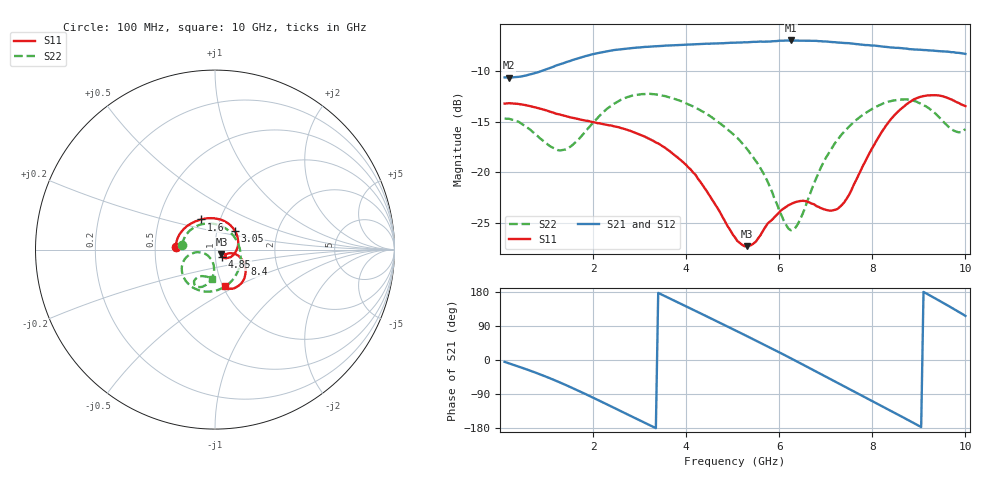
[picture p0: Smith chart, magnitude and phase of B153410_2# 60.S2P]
!  2-Port S-parameters saved by WinCal
! VAR MeasName=S-Parameters (CALIBRATED_DATA) read from VNA (N5245A)
! VAR MeasDate=2016-12-23 10:02:34
! VAR NAME=B153410_2# 60
! VAR FILENAME=B153410_2# 60.S2P
! VAR DATE=2016-12-23 10:02:34
! VAR PHYS_PORTS=1,2
# Hz S DB R 50
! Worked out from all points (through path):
!   199 points, 100 MHz to 10 GHz, reference 50 ohm
!   highest |S21| = -6.94 dB at 6.25 GHz (marker M1); lowest = -10.6 dB at 200 MHz (marker M2)
!   group delay of S21, straight-line fit = 170 ps
!   lowest |S11| = -27.3 dB at 5.3 GHz (marker M3), VSWR 1.09, Z = 53.7 - j2.54 ohm
!   |S11| at or under -10 dB: start of sweep to end of sweep
!   |S22| runs from -25.7 to -12.2 dB; largest |S21 - S12| = 0.0035
!   S11 on the Smith chart (normalised r, x): 100 MHz: 0.64, +0.02; 1.6 GHz: 0.81, +0.28; 3.05 GHz: 1.22, +0.26; 4.85 GHz: 1.08, -0.09; 8.4 GHz: 1.37, -0.23; 10 GHz: 1.02, -0.44
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1e8  -13.20 176.4  -10.60 -4.9  -10.59 -4.8  -14.69 172.4
2e8  -13.16 171.9  -10.62 -9.0  -10.62 -9.0  -14.70 163.7
9e8  -13.75 142.4  -9.96 -39.6  -9.95 -39.7  -16.78 94.6
1.6e9  -14.64 115.2  -8.82 -76.3  -8.84 -76.4  -17.13 0.2
1.75e9  -14.80 109.2  -8.61 -84.8  -8.62 -84.9  -16.44 -18.1
2.35e9  -15.35 81.9  -7.98 -120.1  -7.99 -120.2  -13.54 -72.3
3.05e9  -16.34 43.0  -7.61 -162.1  -7.63 -162.0  -12.26 -112.9
3.4e9  -17.15 21.8  -7.51 177.1  -7.52 177.3  -12.32 -127.7
4.05e9  -19.53 -17.1  -7.34 138.6  -7.35 138.7  -13.28 -148.4
4.85e9  -24.99 -45.9  -7.20 90.7  -7.19 90.7  -15.59 -164.9
5.05e9  -26.46 -44.0  -7.17 78.5  -7.17 78.7  -16.39 -167.8
5.3e9  -27.33 -33.3  -7.13 63.4  -7.11 63.6  -17.65 -170.2
5.8e9  -24.90 -23.4  -7.05 32.8  -7.04 32.9  -21.46 -169.5
6.25e9  -23.15 -29.6  -6.94 4.4  -6.95 4.5  -25.75 -136.1
6.7e9  -23.11 -37.8  -6.96 -24.5  -6.98 -24.4  -21.67 -95.9
7.15e9  -23.78 -30.1  -7.11 -53.6  -7.10 -53.4  -17.47 -93.2
7.5e9  -22.25 -15.6  -7.21 -76.0  -7.24 -76.0  -15.48 -97.6
7.9e9  -18.45 -12.7  -7.40 -101.9  -7.40 -101.7  -14.00 -103.4
8.35e9  -15.04 -24.5  -7.61 -131.1  -7.60 -130.7  -13.00 -110.9
8.4e9  -14.74 -26.0  -7.64 -134.2  -7.62 -134.0  -12.95 -111.9
9.2e9  -12.38 -56.4  -7.92 172.9  -7.90 173.2  -13.61 -123.8
1e10  -13.45 -74.7  -8.28 116.4  -8.27 116.8  -15.72 -95.7
